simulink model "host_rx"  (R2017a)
settings: Solver=FixedStepDiscrete  StartTime=0.0  StopTime=inf  RelTol=1e-3  EnableMultiTasking=on
libraries: c280xlib x1

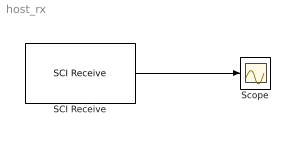
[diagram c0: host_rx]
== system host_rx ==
  SCI Receive : c280xlib/SCI Receive  sciModule=A  dataHead='S'  dataTail='E'  dataType=uint16  dataDim=1  initValue=0  errOption=Output the last received value  errValue=0  sampleTime=0.1  outputStatus=off  postInterrupt=off  numFifo=1
  Scope : Scope
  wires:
  SCI Receive/1 -> Scope/1
